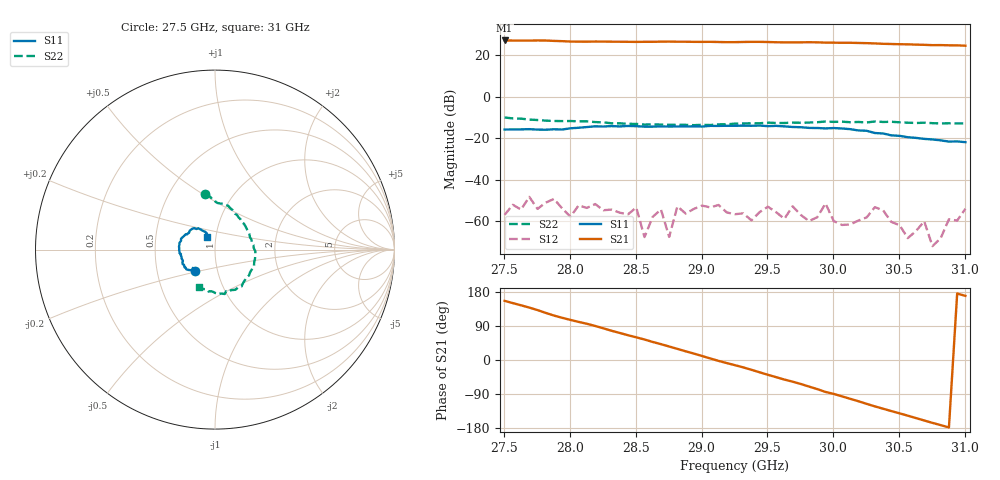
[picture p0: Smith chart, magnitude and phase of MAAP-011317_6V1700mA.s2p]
!Agilent Technologies,E8364C,MY48140145,A.09.42.15
!Agilent E8364C: A.09.42.15
!Date: Friday, June 30, 2023 11:56:05
!Correction: S11(Full 2 Port(1,2))
!S21(Full 2 Port(1,2))
!S12(Full 2 Port(1,2))
!S22(Full 2 Port(1,2))
!S2P File: Measurements: S11, S21, S12, S22:
# Hz S  dB  R 50
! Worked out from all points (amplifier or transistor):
!   57 points, 27.5 GHz to 31 GHz, reference 50 ohm
!   highest |S21| = 27.0 dB at 27.5 GHz (marker M1)
!   |S21| within 3 dB of that: start of sweep to end of sweep
!   unconditionally stable (mu >= 1): start of sweep to end of sweep
!   at 28.07 GHz: K = 8.83, MAG = 26.9 dB, |S12| = -52.3 dB
!   at 29.25 GHz: K = 14.93, MAG = 26.6 dB, |S12| = -56.5 dB
!   at 31 GHz: K = 13.89, MAG = 24.8 dB, |S12| = -53.9 dB
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2.75045e10  -15.81 -133.6  27.01 156.1  -56.80 -158.2  -10.02 100.0
2.769196e10  -15.62 -137.2  26.95 138.3  -48.17 -129.0  -11.02 93.0
2.781694e10  -15.90 -140.5  26.98 124.3  -50.94 -151.6  -11.51 89.2
2.794191e10  -15.80 -138.2  26.67 111.4  -53.74 -130.5  -11.75 83.9
2.812938e10  -14.61 -142.5  26.42 95.6  -53.49 -177.0  -11.86 73.5
2.825435e10  -14.35 -148.3  26.49 83.6  -54.59 -168.9  -12.37 65.6
2.837932e10  -14.31 -154.0  26.40 71.3  -55.79 174.3  -12.82 57.7
2.856679e10  -14.43 -160.3  26.36 54.1  -67.50 -116.5  -13.42 44.6
2.869176e10  -14.31 -164.2  26.44 41.8  -54.22 -158.6  -13.41 37.2
2.875425e10  -14.37 -164.5  26.47 35.6  -67.43 -84.6  -13.53 32.0
2.887922e10  -14.35 -169.2  26.40 22.9  -56.16 -166.3  -13.56 24.1
2.90042e10  -14.36 -172.6  26.32 10.5  -52.37 -173.2  -13.52 15.5
2.925415e10  -14.01 178.4  26.20 -13.7  -56.51 137.8  -12.97 -2.2
2.944161e10  -13.90 169.5  26.34 -32.5  -55.47 -141.7  -12.79 -17.9
2.962908e10  -14.29 159.1  26.10 -51.6  -58.69 151.6  -12.66 -33.2
2.987902e10  -15.07 149.2  26.10 -76.8  -57.94 168.2  -12.30 -49.8
3.012898e10  -15.62 133.9  25.90 -102.4  -61.42 74.3  -12.30 -68.3
3.031644e10  -17.48 124.6  25.59 -122.4  -53.12 164.5  -11.93 -77.7
3.044141e10  -18.60 120.4  25.31 -134.8  -60.20 157.8  -12.08 -85.4
3.069136e10  -20.30 120.5  24.91 -159.7  -59.94 160.5  -12.52 -98.7
3.081634e10  -21.01 117.0  24.78 -171.9  -68.00 15.7  -12.90 -103.6
3.10038e10  -21.89 122.8  24.49 169.3  -53.88 -132.1  -12.88 -112.8
